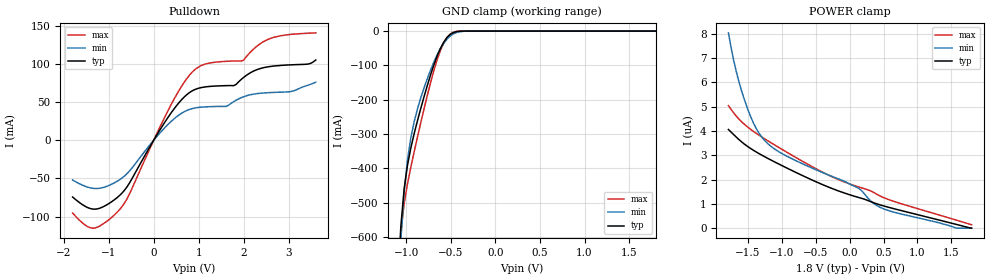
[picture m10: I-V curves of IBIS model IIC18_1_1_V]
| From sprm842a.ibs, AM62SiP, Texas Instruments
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|   Model IIC18_1_1_V
[Model]  IIC18_1_1_V
Model_type I/O_open_drain
Polarity   Non-Inverting
Enable   Active-High
Vinl =  0.540V
Vinh =  1.260V
Vmeas =  0.900V
Cref =  50.000pF
Rref =  1.000M
Vref =  0.0V
C_comp   8.659pF   8.515pF   8.754pF
[Model Spec]
Vinh   1.260V   1.134V   1.386V
Vinl   0.540V   0.486V   0.594V
Vmeas   0.900V   NA   NA
Vref   0.0V   NA   NA
Cref   50.000pF   NA   NA
Rref   1.000M   NA   NA
[Temperature Range]   25.000   0.125k   -40.000
[Voltage Range]   1.800V   1.620V   1.980V
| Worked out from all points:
|   slope of the pulldown table from 0 to 0.27 V, typ, clamps not added: 10.5 ohm
|   GND clamp passes 1 mA (typ) near -0.42 V on its own axis
[Pulldown]
|Voltage   I(typ)   I(min)   I(max)
-1.8V     -74.43mA   -52.12mA   -95.36mA
-1.525V   -86.51mA   -60.23mA   -111.1mA
-1.305V   -90.39mA   -63.27mA   -115.1mA
-755mV    -72.29mA   -51.71mA   -90.8mA
-535mV    -55.85mA   -40.22mA   -70.21mA
400mV     36.93mA    25.37mA    48.14mA
950mV     67.4mA     42.7mA     94.32mA
1.775V    71.64mA    50.63mA    104mA
1.995V    82.32mA    57.1mA     105mA
2.325V    93.33mA    61.41mA    124.9mA
2.655V    97.31mA    62.78mA    134.8mA
3.6V      105.3mA    76.2mA     140.9mA
[GND_clamp]
|Voltage   I(typ)   I(min)   I(max)
-1.8V     -13.06A    -12.03A    -14.07A
-1.097V   -750.9mA   -811mA     -744.1mA
-1.06V    -568.7mA   -607.9mA   -587.9mA
-1.023V   -459.9mA   -469mA     -502.8mA
-986mV    -391.5mA   -376.2mA   -445.5mA
-912mV    -300.2mA   -265.5mA   -353.1mA
-801mV    -192.3mA   -166.3mA   -227.7mA
-653mV    -72.66mA   -69.43mA   -83.58mA
-579mV    -32.26mA   -35.8mA    -34.59mA
-505mV    -9.385mA   -14.2mA    -8.27mA
-320mV    -33.94uA   -278.5uA   -6.542uA
1.8V      0A         0A         0A
[POWER_clamp]
|Voltage   I(typ)   I(min)   I(max)
-1.789V   4.06uA     8.036uA    5.043uA
-1.678V   3.76uA     6.495uA    4.626uA
-1.604V   3.573uA    5.732uA    4.404uA
-1.493V   3.337uA    4.814uA    4.134uA
-1.345V   3.08uA     3.938uA    3.84uA
-1.16V    2.802uA    3.365uA    3.514uA
-383mV    1.773uA    2.269uA    2.282uA
135mV     1.261uA    1.635uA    1.696uA
320mV     1.081uA    1.098uA    1.522uA
505mV     912.7nA    791.1nA    1.254uA
1.578V    151.7nA    0A         328nA
1.8V      0A         0A         138.8nA
[Ramp]
| variable   typ   min   max
dV/dt_r   0.891/0.444n   0.740/0.440n   1.022/0.471n
dV/dt_f   0.231/21.099n   91.039m/16.097n   0.456/15.705n
R_load = 50.000
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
